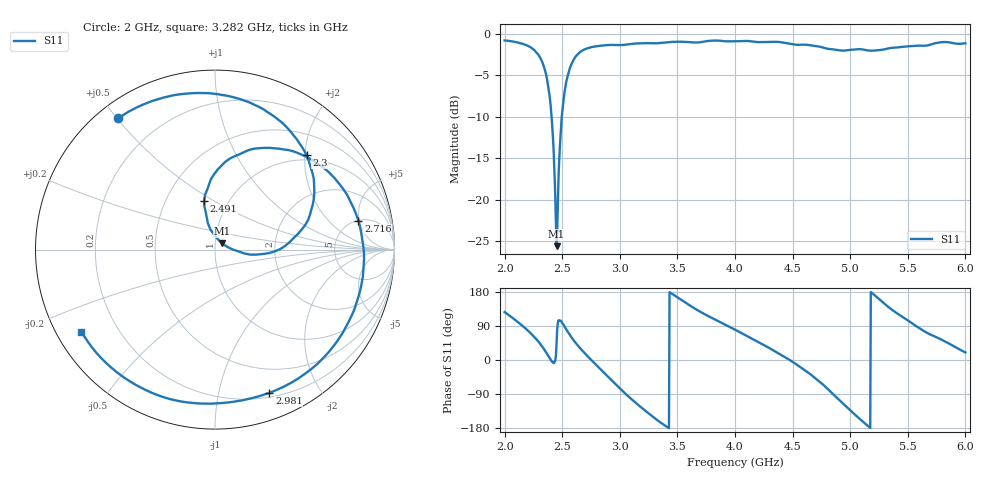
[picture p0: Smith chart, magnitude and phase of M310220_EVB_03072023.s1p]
# Hz S RI R 50
! CMT, M5090, 19127454, 21.2.4/2
! Date: 3/7/2023 4:24:05 PM
! Data: Format (Calibration Info)
! Freq	S11:Re/Im(F2)
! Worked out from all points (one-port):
!   800 points, 2 GHz to 6 GHz, reference 50 ohm
!   lowest |S11| = -25.6 dB at 2.451 GHz (marker M1), VSWR 1.11, Z = 54 + j3.73 ohm
!   |S11| at or under -10 dB: 2.407 GHz to 2.496 GHz (88.8 MHz wide, 3.62 % of centre)
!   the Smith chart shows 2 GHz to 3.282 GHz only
!   S11 on the Smith chart (normalised r, x): 2 GHz: 0.06, +0.50; 2.3 GHz: 0.89, +2.03; 2.491 GHz: 0.77, +0.45; 2.716 GHz: 5.05, +4.87; 2.981 GHz: 0.24, -1.42; 3.282 GHz: 0.07, -0.28
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2e9  -0.5407 0.7309
2.170213e9  0.0559 0.8591
2.300375e9  0.5098 0.5269
2.390488e9  0.4186 0.0441
2.450563e9  0.0395 0.0345
2.490613e9  -0.0615 0.2709
2.500626e9  -0.0425 0.336
2.585732e9  0.356 0.5626
2.715895e9  0.7994 0.1614
2.841051e9  0.7531 -0.3848
2.981227e9  0.3032 -0.798
3.001252e9  0.2179 -0.8245
3.126408e9  -0.2955 -0.8193
3.281602e9  -0.7438 -0.4581
3.501877e9  -0.8643 0.2283
3.757196e9  -0.4177 0.7983
4.002503e9  0.1612 0.8844
4.312891e9  0.7803 0.431
4.503129e9  0.8585 -0.0819
4.643304e9  0.6975 -0.4893
4.788486e9  0.2556 -0.7737
5.003755e9  -0.5524 -0.5766
5.108886e9  -0.764 -0.2453
5.229036e9  -0.7709 0.1843
5.364205e9  -0.5513 0.6084
5.50438e9  -0.1977 0.8145
5.769712e9  0.4789 0.7425
6e9  0.8218 0.2978
